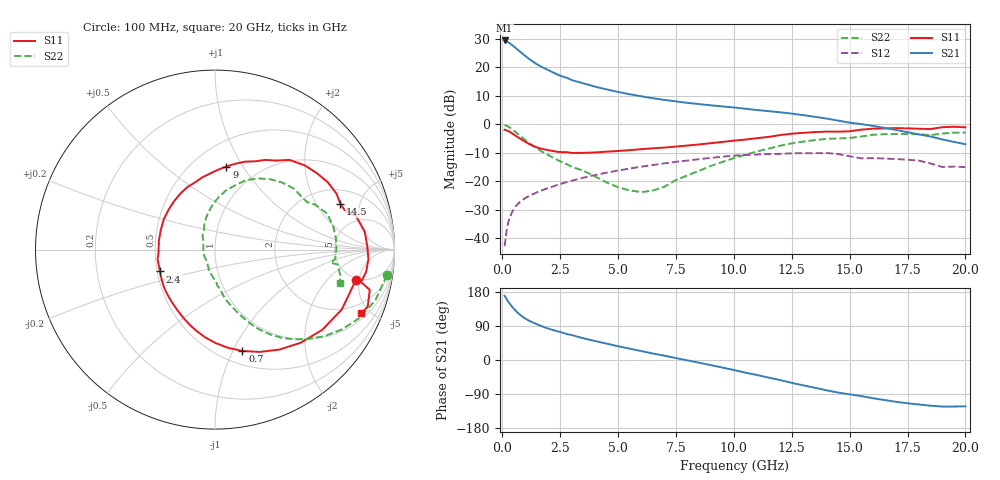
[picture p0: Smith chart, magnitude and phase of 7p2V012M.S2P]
! Infineon Technologies  Discrete & RF Semiconductors
! bfp620
! VCE =  2.0 V,  IC =  12 mA
! Common Emitter S-Parameters:  Sep 2002
# GHz  S  MA  R  50
!  f  S11  S21  S12  S22
! GHz  MAG  ANG  MAG  ANG  MAG  ANG  MAG  ANG
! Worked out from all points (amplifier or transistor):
!   59 points, 100 MHz to 20 GHz, reference 50 ohm
!   highest |S21| = 29.4 dB at 100 MHz (marker M1)
!   |S21| within 3 dB of that: start of sweep to 630.5 MHz
!   unconditionally stable (mu >= 1): 3.855 GHz to 10.51 GHz; 17.13 GHz to end of sweep
!   at 1 GHz: K = 0.55, MSG = 24.9 dB, |S12| = -25.8 dB
!   at 5.5 GHz: K = 1.05, MAG = 11.7 dB, |S12| = -15.5 dB
!   at 20 GHz: K = 1.31, MAG = 0.7 dB, |S12| = -15.0 dB
!   S11 on the Smith chart (normalised r, x): 100 MHz: 4.77, -4.53; 700 MHz: 0.63, -1.09; 2.4 GHz: 0.52, -0.14; 9 GHz: 0.72, +0.85; 14.5 GHz: 2.89, +3.27; 20 GHz: 1.31, -4.41
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0.1  0.8033 -12.1  29.62 169.6  0.0073 76.4  0.969 -8.4
0.2  0.7812 -25.3  28.4 159.3  0.0151 74.7  0.937 -17.6
0.3  0.7463 -36.8  26.8 150.4  0.0219 70.8  0.8899 -25.4
0.4  0.705 -47.4  25.03 142.5  0.0277 66.9  0.8348 -32.2
0.5  0.6626 -57.2  23.22 135.3  0.0328 63.5  0.7769 -38.4
0.6  0.6221 -66.4  21.48 128.7  0.0373 60.6  0.7198 -43.8
0.7  0.5849 -74.9  19.85 122.8  0.0413 58.2  0.6657 -48.7
0.8  0.5509 -82.7  18.35 117.6  0.0449 56.1  0.6155 -52.9
1  0.4919 -96.4  15.75 109.1  0.0511 53.1  0.528 -59.6
1.3  0.4245 -113.3  12.77 99.6  0.0591 50.3  0.4271 -66.4
1.8  0.3656 -136.1  9.732 87.0  0.0718 47.6  0.3186 -74.7
2.4  0.3298 -158.3  7.427 75.5  0.087 44.6  0.2356 -81.6
3  0.3152 -176.8  5.976 65.7  0.1027 41.0  0.1802 -87.5
3.5  0.3165 171.2  5.237 57.3  0.1161 37.7  0.1539 -94.7
5  0.341 139.3  3.703 36.3  0.1551 26.3  0.0787 -127.2
7  0.3912 106.4  2.683 11.4  0.2067 9.4  0.0804 143.8
9  0.4673 82.2  2.159 -13.5  0.258 -10.3  0.1863 105.1
10.5  0.5405 65.5  1.877 -33.4  0.2899 -27.8  0.2933 85.9
13.5  0.7322 30.8  1.355 -73.3  0.3121 -62.1  0.5296 44.8
14.5  0.7435 19.9  1.162 -85.9  0.3019 -77.0  0.5646 31.5
17  0.8563 -3.5  0.8 -110.2  0.2461 -93.4  0.6766 5.3
20  0.8881 -23.6  0.448 -122.3  0.178 -104.6  0.7191 -15.1
